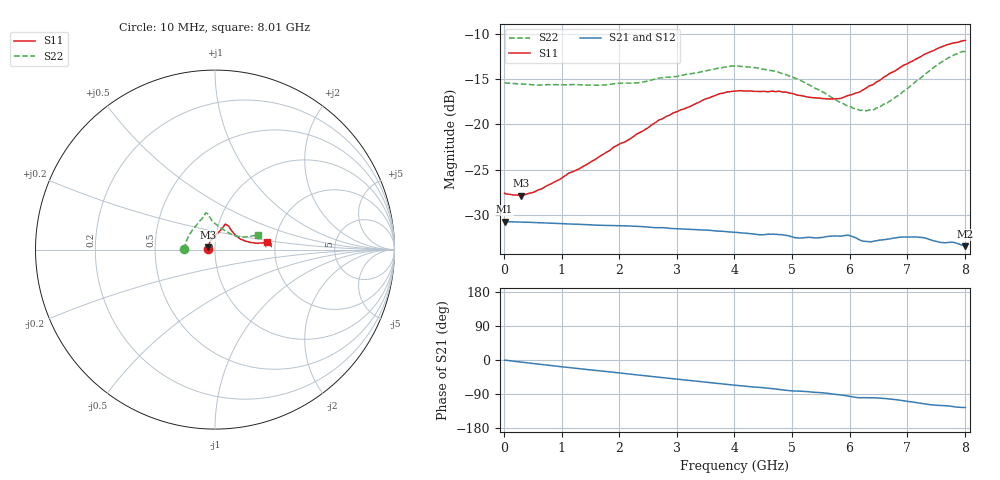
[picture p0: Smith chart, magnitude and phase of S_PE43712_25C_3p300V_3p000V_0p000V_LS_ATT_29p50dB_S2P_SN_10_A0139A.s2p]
! DEVICE ID: PE43712
! File Path: z:\PE43713\PE43713_CHAR_NOM_04292014\AMB\3p300\LS_ATT_29p50dB\PE43713_AMB_3p300V_3p000V_0p000V_LS_ATT_29p50dB_S2P_SN_10_A0139A.s2p
! Serial: 10
! Lot: A0139A
! Temp: 25C
! VDD: 3.300
! VSS: 0.000
! Control_Hi: 3.000
! Control_Lo: 0.000
! Attenuation Step: 29.50dB
! Port 1: RF1
! Port 2: RF2
! ThroughPath:1-2
! IDD: 0.000145657
! ISS: -8.72e-008
#  Hz  S  RI  R  50
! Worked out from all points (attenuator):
!   801 points, 10 MHz to 8.01 GHz, reference 50 ohm
!   highest |S21| = -30.76 dB at 10 MHz (marker M1); lowest = -33.5 dB at 8 GHz (marker M2)
!   lowest |S11| = -27.9 dB at 290 MHz (marker M3), VSWR 1.08, Z = 46.3 + j1.23 ohm
!   |S11| at or under -10 dB: start of sweep to end of sweep
!   |S22| runs from -18.5 to -11.9 dB; largest |S21 - S12| = 0.00011
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1e7  -0.0416 0.000906  0.029 -0.000138  0.0289 -0.00012  -0.1704 0.00123
2.9e8  -0.0381 0.0133  0.0287 -0.00271  0.0287 -0.00272  -0.1663 0.0192
6.5e8  -0.0337 0.0281  0.0279 -0.00582  0.0279 -0.00582  -0.1601 0.0411
1.35e9  -0.021 0.054  0.0256 -0.0112  0.0256 -0.0112  -0.1444 0.081
2.28e9  0.00949 0.0869  0.0212 -0.0171  0.0212 -0.0171  -0.1071 0.1314
2.68e9  0.0251 0.1023  0.0188 -0.019  0.0188 -0.019  -0.0875 0.1579
3.5e9  0.0484 0.1297  0.0136 -0.0221  0.0136 -0.0221  -0.0594 0.1886
3.74e9  0.0533 0.1379  0.0119 -0.0227  0.0119 -0.0227  -0.0556 0.1979
4.01e9  0.0582 0.1415  0.0101 -0.0232  0.0101 -0.0232  -0.0531 0.2038
4.75e9  0.072 0.1345  0.00538 -0.024  0.00543 -0.024  -0.0348 0.1923
5.09e9  0.082 0.1201  0.00328 -0.0233  0.00329 -0.0233  -0.0257 0.1768
5.35e9  0.0911 0.1073  0.00213 -0.0235  0.00212 -0.0235  -0.0174 0.1616
5.81e9  0.1136 0.0799  -0.000723 -0.024  -0.000695 -0.0241  0.0153 0.1329
5.99e9  0.1269 0.0704  -0.00246 -0.0241  -0.00248 -0.0241  0.0319 0.1223
6.17e9  0.1386 0.0602  -0.00379 -0.0227  -0.00371 -0.0227  0.0504 0.1086
6.4e9  0.1574 0.0521  -0.00373 -0.0222  -0.00365 -0.0221  0.0761 0.0926
6.68e9  0.1852 0.0435  -0.00504 -0.0227  -0.00504 -0.0226  0.1088 0.0775
7.2e9  0.2315 0.0358  -0.00941 -0.0218  -0.00938 -0.0217  0.1631 0.0698
7.56e9  0.2637 0.0375  -0.0111 -0.0193  -0.0111 -0.0193  0.2043 0.0755
7.81e9  0.2801 0.0406  -0.0121 -0.0185  -0.0121 -0.0186  0.2285 0.0816
8e9  0.2882 0.0427  -0.0122 -0.0173  -0.0122 -0.0173  0.2395 0.0829
8.01e9  0.2886 0.0432  -0.0122 -0.0173  -0.0122 -0.0173  0.2401 0.0828
